DATA_BLOCK "Demo2"
VERSION : 0.1


  STRUCT
   str1 : STRING  [254 ] := '456 abcdefgh$R';	//write $$ to insert one single $; write $R to insert <CR> (0d hex)
  END_STRUCT ;
BEGIN
   str1 := '456 abcdefgh$R';
END_DATA_BLOCK

